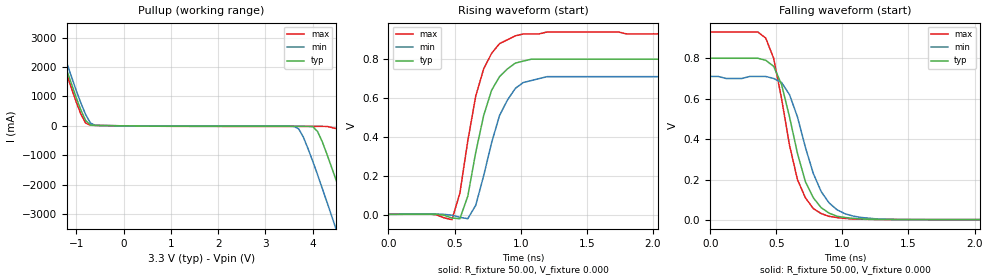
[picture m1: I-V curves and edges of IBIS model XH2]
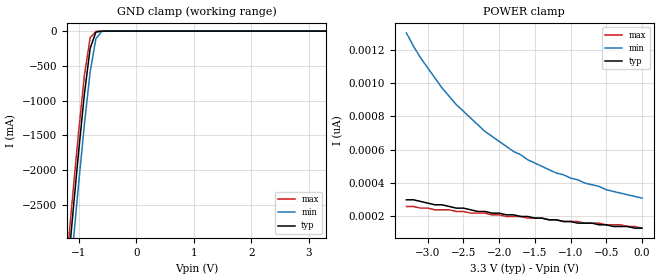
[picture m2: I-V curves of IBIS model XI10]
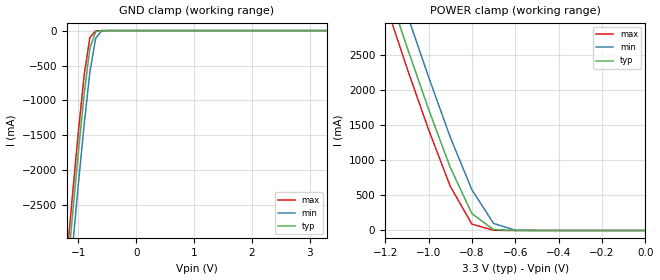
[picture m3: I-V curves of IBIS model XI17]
|   * 9db106b.ibs * IBIS 2.1 Model file
| Rev History
| Rev No.  Description
| 1.0   Initial release with Updated Parasitic Parameters  Dec 2, 2003
| 1.1   Integrated Circuit Systems => Integrated Device Technology
| 1.2   Updated XH2 and XIO3 models to include Vmeas, Vref etc
[IBIS Ver]   2.1
[Comment char]  |_char
[File name]   9db106b.ibs
[Date]   March 23, 2012
[File Rev]   1.2
[Source]   Originated at Integrated Device Technology, Inc.
[Disclaimer] (C) Copyright Integrated Device Technology, Inc. 2010
   All rights reserved
IDT hereby grants the user of this IBIS model a non-exclusive,
nontransferable license to use this IBIS model under the following terms.
Before using this IBIS model, the user should read this license.
If the user does not accept these terms, the IBIS model should be
returned to IDT within 30 days.
   The user is granted this license only to use the IBIS model and
is not granted rights to sell, load, rent, lease or license the IBIS
model in whole or in part, or in modified form to anyone other than
user. User may modify the IBIS model to suit its specific
applications but rights to derivative works and such modifications
shall belong to IDT.
   This IBIS model is provided on an "AS IS" basis and IDT makes
absolutely no warranty with respect to the information contained
herein. IDT DISCLAIMS AND CUSTOMER WAIVES ALL WARRANTIES, EXPRESS
OR IMPLIED, INCLUDING WARRANTIES OF MERCHANTABILITY OR FITNESS FOR
A PARTICULAR PURPOSE. The entire risk as to quality and performance
is with the Customer. ACCORDINGLY, IN NO EVENT SHALL THE COMPANY BE
LIABLE FOR ANY DAMAGES, WHETHER IN CONTRACT OR TORT,INCLUDING ANY
LOST PROFITS OR OTHER INCIDENTAL, CONSEQUENTIAL, EXEMPLARY, OR
PUNITIVE DAMAGES ARISING OUT OF THE USE OR APPLICATION OF THE IBIS
model provided in this package. Further, IDT reserves the right to
make changes without notice to any product herein to improve
reliability, function, or design. IDT does not convey any license
under patent rights or any other intellectual property rights,
including those of third parties.
   IDT is not obligated to provide maintenance or support
for the licensed IBIS model.
|   COMPONENT: IDT9DB106B
[Component]   IDT9DB106B
[Manufacturer]  IDT
[Package]
| variable   typ   min   max
R_pkg   81.1m   62.2m   100.0m
L_pkg   6.7nH   4.9nH   8.5nH
C_pkg   0.53pF  0.21pF  0.85pF
[Pin]   signal_name   model_name   R_pin   L_pin   C_pin
  1   PLL_BW   XI29
  2   CLK_INT   XI4
  3   CLK_INC   XI4
  4   OE1B   XI20
  5   PCIEXT0   XH2
  6   PCIEXC0   XH2
  7   VDD   POWER
  8   GND   GND
  9   PCIEXT1   XH2
 10   PCIEXC1   XH2
 11   PCIEXT2   XH2
 12   PCIEXC2   XH2
 13   VDD   POWER
 14   SMBDAT   XIO3
 15   SMBCLK   XI10
 16   VDD   POWER
 17   PCIEXC3   XH2
 18   PCIEXT3   XH2
 19   PCIEXC4   XH2
 20   PCIEXT4   XH2
 21   GND   GND
 22   VDD   POWER
 23   PCIEXC5   XH2
 24   PCIEXT5   XH2
 25   OE4B   XI20
 26   IREF   XI17
 27   GNDA   GND
 28   VDDA   POWER
|* Either 3.3V or 2.5V
|** All model are simulated with typical corner process
[Diff Pin]   inv_pin   vdiff   tdelay_typ
5   6   NA   NA
9   10   NA   NA
11   12   NA   NA
18   17   NA   NA
20   19   NA   NA
24   23   NA   NA
2   3   NA   NA
| Models and submodels in the file (7): XH2 (Open_source), XI10 (Input), XI17 (Input), XI20 (Input), XI29 (Input), XI4 (Input), XIO3 (I/O_open_drain)
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|   Model XH2
[Model]   XH2
Model_type   Open_source
Polarity   Inverting
Vmeas = 0.35V
Cref =   2.00pF
Rref =  500
Vref =   0.0V
C_comp   3.40pF   2.85pF   3.95pF
[Temperature Range]   27.00   70.00   0.000
[Voltage Range]   3.30V   3.00V   3.70V
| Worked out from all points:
|   slope of the pullup table from 0 to 0.495 V, typ, clamps not added: 55.1 ohm
|   rising waveform, R_fixture 50.00, V_fixture 0.000: 20-80 % time 163ps typ, 186ps min, 160ps max; typ from 0.002 V to 0.8 V
|   falling waveform, R_fixture 50.00, V_fixture 0.000: 20-80 % time 190ps typ, 210ps min, 172ps max; typ from 0.8 V to 0.002 V
[Pullup]
| voltage   I(typ)   I(min)   I(max)
-3.3V     12.12A     12.35A     11.98A
-1.7V     4.26A      4.5A       4.11A
-1.5V     3.29A      3.54A      3.14A
-900mV    530mA      770mA      390mA
-700mV    28.34mA    96.53mA    20.48mA
3.7V      -16.09mA   -100mA     -18.73mA
4.1V      -190mA     -1.66A     -18.77mA
4.5V      -1.88A     -3.55A     -97.21mA
4.7V      -2.83A     -4.52A     -820mA
4.9V      -3.79A     -5.49A     -1.73A
5.3V      -5.74A     -7.45A     -3.64A
6.6V      -12.15A    -13.87A    -10.03A
[Ramp]
| variable   typ   min   max
dV/dt_r   0.48/0.16n   0.42/0.17n   0.56/0.16n
dV/dt_f   0.48/0.18n   0.42/0.21n   0.56/0.17n
R_load = 50.00
[Rising Waveform]
R_fixture = 50.00
V_fixture = 0.000
V_fixture_min = 0.000
V_fixture_max = 0.000
| time   V(typ)   V(min)   V(max)
0s        1.72mV     1.4mV      2.09mV
480ps     -17.54mV   -2.8mV     -26.08mV
540ps     -21.03mV   -14.08mV   110mV
600ps     94.95mV    -20.91mV   380mV
660ps     320mV      47.82mV    610mV
720ps     510mV      200mV      750mV
840ps     710mV      510mV      880mV
960ps     780mV      650mV      920mV
1.2ns     800mV      710mV      940mV
3ns       800mV      710mV      930mV
[Falling Waveform]
R_fixture = 50.00
V_fixture = 0.000
V_fixture_min = 0.000
V_fixture_max = 0.000
| time   V(typ)   V(min)   V(max)
0s        800mV      710mV      930mV
420ps     790mV      710mV      900mV
480ps     760mV      700mV      800mV
540ps     670mV      680mV      600mV
660ps     330mV      510mV      200mV
720ps     190mV      360mV      110mV
840ps     60.55mV    140mV      31.59mV
960ps     18.32mV    50.26mV    11.75mV
1.14ns    5.19mV     12.59mV    3.78mV
3ns       1.77mV     1.45mV     2.15mV
|   Model XI10
[Model]   XI10
Model_type   Input
Polarity   Inverting
Vinl =   0.80V
Vinh =   2.00V
C_comp   5.50pF   5.00pF   6.00pF
[Temperature Range]   27.00   70.00   0.000
[Voltage Range]   3.30V   3.00V   3.70V
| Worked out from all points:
|   GND clamp passes 1 mA (typ) near -0.60 V on its own axis
[GND_clamp]
| voltage   I(typ)   I(min)   I(max)
-3.3V     -24.05A    -24.49A    -23.79A
-1.2V     -3.55A     -4.02A     -3.26A
-1.1V     -2.63A     -3.1A      -2.34A
-1V       -1.74A     -2.2A      -1.45A
-900mV    -910mA     -1.35A     -640mA
-800mV    -250mA     -590mA     -96.82mA
-700mV    -14.58mA   -110mA     -3.87mA
-600mV    -880uA     -5.84mA    -450uA
-500mV    -88.5uA    -350uA     -45.09uA
3.3V      130pA      340pA      120pA
[POWER_clamp]
| voltage   I(typ)   I(min)   I(max)
-3.3V     300pA      1.3nA      260pA
-3.1V     290pA      1.15nA     250pA
-2.9V     270pA      1.03nA     240pA
-2.8V     270pA      970pA      240pA
-2.6V     250pA      870pA      230pA
-2.2V     230pA      710pA      220pA
-1.8V     210pA      590pA      200pA
-1.2V     180pA      460pA      180pA
-900mV    160pA      420pA      170pA
-500mV    150pA      360pA      150pA
-300mV    140pA      340pA      150pA
0V        130pA      310pA      130pA
|   Model XI17
[Model]   XI17
Model_type   Input
Vinl =   0.80V
Vinh =   2.00V
C_comp   5.50pF   5.00pF   6.00pF
[Temperature Range]   27.00   70.00   0.000
[Voltage Range]   3.30V   3.00V   3.70V
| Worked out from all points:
|   GND clamp passes 1 mA (typ) near -0.60 V on its own axis
|   POWER clamp passes 1 mA (typ) near -0.61 V on its own axis
[GND_clamp]
| voltage   I(typ)   I(min)   I(max)
-3.3V     -24.05A    -24.48A    -23.79A
-1.2V     -3.55A     -4.02A     -3.26A
-1.1V     -2.63A     -3.1A      -2.34A
-1V       -1.74A     -2.2A      -1.45A
-900mV    -910mA     -1.35A     -640mA
-800mV    -250mA     -590mA     -96.82mA
-700mV    -14.58mA   -110mA     -3.87mA
-600mV    -880uA     -5.82mA    -450uA
-500mV    -88.5uA    -350uA     -45.09uA
3.3V      130pA      240nA      110pA
[POWER_clamp]
| voltage   I(typ)   I(min)   I(max)
-3.3V     24.04A     24.47A     23.78A
-1.2V     3.54A      4.01A      3.25A
-1.1V     2.62A      3.09A      2.32A
-1V       1.73A      2.19A      1.44A
-900mV    900mA      1.33A      630mA
-800mV    240mA      580mA      90.95mA
-700mV    12.08mA    100mA      1.95mA
-600mV    280uA      4.78mA     32.65uA
0V        130pA      310pA      130pA
